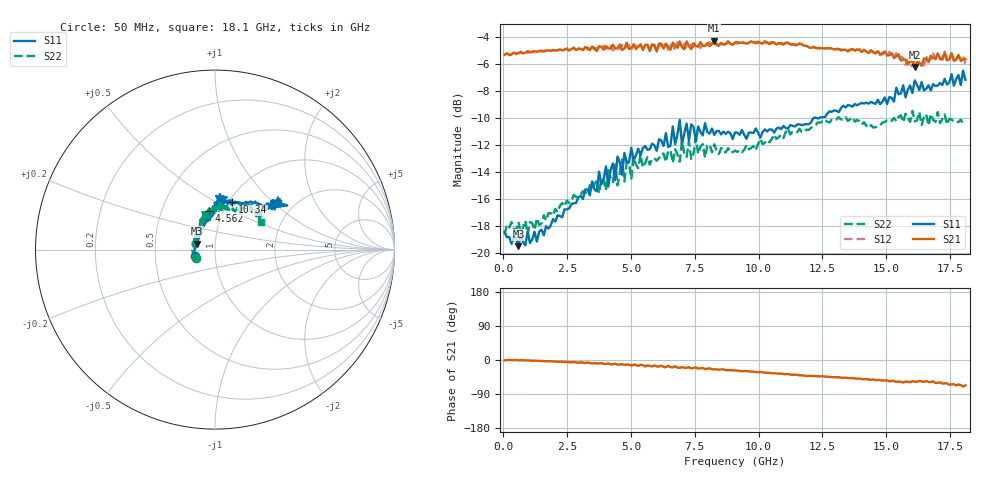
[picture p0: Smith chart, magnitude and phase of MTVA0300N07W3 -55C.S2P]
! Network Analyzer HP8720D.06.14 Serial No. US36140669
!  7 Jul 2005  11:47:41
! Frequency  S11  S21  S12  S22
# HZ  S  DB R 50
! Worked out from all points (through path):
!   201 points, 50 MHz to 18.1 GHz, reference 50 ohm
!   highest |S21| = -4.29 dB at 8.263 GHz (marker M1); lowest = -6.2 dB at 16.11 GHz (marker M2)
!   group delay of S21, straight-line fit = 10.7 ps
!   lowest |S11| = -19.5 dB at 591.5 MHz (marker M3), VSWR 1.24, Z = 40.8 + j2.8 ohm
!   |S11| at or under -10 dB: start of sweep to 12.41 GHz
!   |S22| runs from -18.7 to -9.5 dB; largest |S21 - S12| = 0.039
!   S11 on the Smith chart (normalised r, x): 50 MHz: 0.79, -0.06; 4.562 GHz: 0.85, +0.38; 10.34 GHz: 1.04, +0.59; 18.1 GHz: 1.65, +1.07
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5e7  -18.48 -162.6  -5.34 -0.8  -5.33 -0.7  -18.65 -157.3
5.915e8  -19.53 161.3  -5.24 -0.8  -5.18 -0.8  -17.74 166.9
9.525e8  -18.43 151.8  -5.08 -1.1  -5.19 -0.9  -18.65 156.5
3.1185e9  -16.02 109.3  -5.01 -6.9  -5.00 -7.5  -15.44 119.5
4.5625e9  -13.32 99.2  -4.59 -11.9  -4.90 -12.4  -14.12 99.8
6.09675e9  -11.61 85.5  -4.56 -17.5  -4.49 -16.9  -13.00 93.1
6.548e9  -12.07 80.7  -4.97 -18.6  -4.64 -20.2  -12.43 91.7
6.63825e9  -10.65 85.0  -4.45 -19.6  -4.63 -17.5  -13.36 88.0
6.7285e9  -11.96 89.5  -4.67 -16.5  -4.98 -18.4  -12.35 85.1
6.909e9  -10.17 85.0  -4.36 -20.9  -4.61 -18.6  -13.27 84.4
6.99925e9  -11.99 85.0  -4.79 -18.5  -4.87 -21.5  -11.78 84.1
7.17975e9  -10.44 88.8  -4.36 -20.4  -4.80 -19.4  -12.92 79.2
7.27e9  -11.69 83.8  -4.72 -19.2  -4.77 -22.2  -11.77 82.9
7.36025e9  -10.50 77.3  -4.92 -22.1  -4.58 -20.1  -13.07 87.8
7.54075e9  -11.76 79.6  -4.70 -19.5  -4.44 -22.9  -11.49 85.7
8.26275e9  -11.28 82.2  -4.29 -24.6  -4.52 -25.8  -11.98 73.9
9.075e9  -11.10 78.0  -4.45 -27.5  -4.41 -27.5  -12.45 71.0
1.03385e10  -11.03 70.3  -4.44 -33.4  -4.47 -33.9  -11.66 58.7
1.21435e10  -10.03 57.5  -4.78 -42.2  -4.73 -42.2  -10.63 56.5
1.512175e10  -8.47 37.5  -5.38 -56.2  -5.12 -55.5  -10.19 45.0
1.61145e10  -7.24 35.8  -6.25 -56.8  -5.74 -56.6  -10.28 41.7
1.81e10  -7.20 36.8  -5.68 -66.9  -6.01 -67.3  -10.43 30.7
